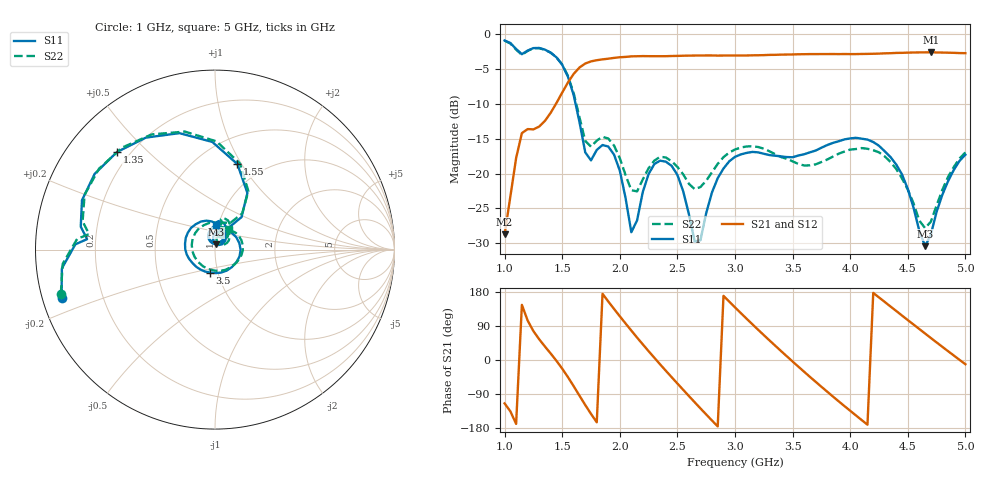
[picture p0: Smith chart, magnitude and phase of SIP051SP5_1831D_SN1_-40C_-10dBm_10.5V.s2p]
# GHz  S  dB  R  50
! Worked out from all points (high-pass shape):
!   81 points, 1 GHz to 5 GHz, reference 50 ohm
!   highest |S21| = -2.65 dB at 4.7 GHz (marker M1); lowest = -28.7 dB at 1 GHz (marker M2)
!   |S21| within 3 dB of the highest: 1.605 GHz to end of sweep
!   lowest |S11| = -30.4 dB at 4.65 GHz (marker M3), VSWR 1.06, Z = 50.5 + j3 ohm
!   |S11| at or under -10 dB: 1.616 GHz to end of sweep
!   |S22| runs from -27.8 to -1.0 dB; largest |S21 - S12| = 0.002
!   S11 on the Smith chart (normalised r, x): 1 GHz: 0.06, -0.15; 1.35 GHz: 0.15, +0.40; 1.55 GHz: 0.76, +0.96; 3.5 GHz: 0.92, -0.24; 5 GHz: 0.97, +0.27
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1  -0.95 -162.6  -28.73 -114.5  -28.80 -114.5  -0.97 -164.0
1.15  -2.91 175.3  -14.22 145.5  -14.21 145.5  -3.01 173.0
1.35  -2.26 135.2  -12.47 35.6  -12.47 35.6  -2.29 132.3
1.55  -6.15 75.3  -6.96 -45.3  -6.95 -45.3  -6.03 73.8
1.7  -16.97 58.3  -4.26 -118.8  -4.26 -118.8  -15.33 60.2
1.85  -15.92 83.0  -3.66 174.6  -3.65 174.6  -14.75 74.8
2.05  -23.51 49.0  -3.31 96.4  -3.31 96.4  -20.22 49.7
2.1  -28.41 70.5  -3.23 77.7  -3.24 77.7  -22.40 60.2
2.35  -18.16 87.8  -3.21 -11.4  -3.19 -11.4  -17.60 71.4
2.5  -20.20 50.3  -3.16 -62.1  -3.16 -62.0  -19.05 48.4
2.65  -29.74 51.0  -3.11 -111.4  -3.10 -111.5  -22.24 53.1
2.85  -20.66 86.4  -3.12 -175.3  -3.11 -175.3  -18.62 61.9
3  -17.62 45.5  -3.11 138.9  -3.10 138.9  -16.56 38.9
3.25  -17.17 -30.6  -3.05 65.7  -3.05 65.8  -16.45 -11.6
3.5  -17.67 -102.2  -2.96 -4.0  -2.95 -4.0  -18.26 -76.4
3.7  -16.71 -149.0  -2.90 -57.5  -2.90 -57.5  -18.69 -143.5
3.85  -15.62 179.5  -2.89 -96.4  -2.88 -96.3  -17.58 168.9
4.05  -14.89 137.9  -2.90 -146.3  -2.88 -146.4  -16.50 114.5
4.35  -17.64 76.3  -2.78 141.2  -2.78 141.2  -18.36 49.7
4.65  -30.40 79.4  -2.66 69.9  -2.66 69.8  -27.82 56.1
4.7  -28.76 109.9  -2.65 58.1  -2.65 58.1  -26.90 74.8
5  -17.32 87.6  -2.77 -11.1  -2.78 -11.2  -16.98 55.9
